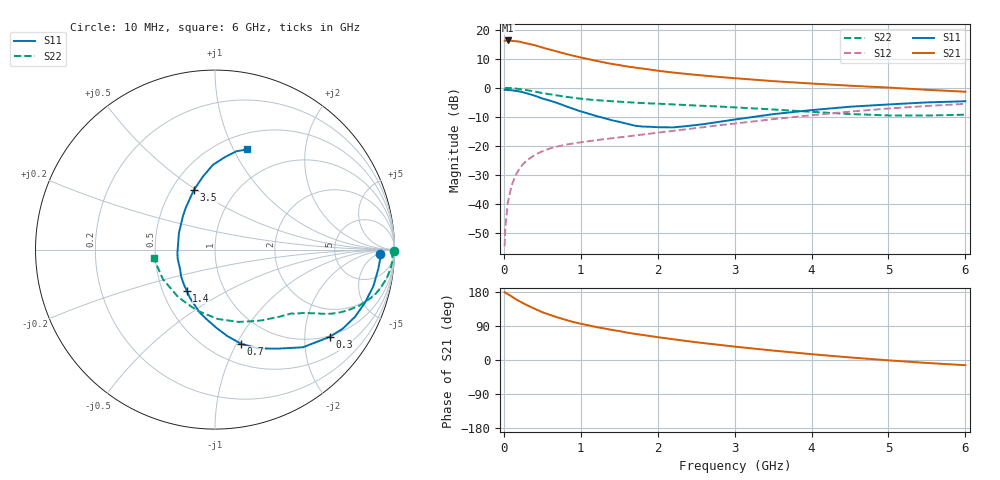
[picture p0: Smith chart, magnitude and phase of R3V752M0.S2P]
! SIEMENS Small Signal Semiconductors
! BFR181
! Si NPN RF Bipolar Junction Transistor in SOT23
! VCE = 0.75 V  IC = 2 mA
! Common Emitter S-Parameters:  May  1996
# GHz  S  MA  R  50
!  f  S11  S21  S12  S22
! GHz  MAG  ANG  MAG  ANG  MAG  ANG  MAG  ANG
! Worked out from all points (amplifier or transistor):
!   36 points, 10 MHz to 6 GHz, reference 50 ohm
!   highest |S21| = 16.3 dB at 50 MHz (marker M1)
!   |S21| within 3 dB of that: start of sweep to 578.3 MHz
!   unconditionally stable (mu >= 1): 1.459 GHz to 3.723 GHz
!   at 250 MHz: K = 0.24, MSG = 20.9 dB, |S12| = -26.3 dB
!   at 1.4 GHz: K = 0.98, MSG = 12.8 dB, |S12| = -17.4 dB
!   at 6 GHz: K = 0.92, MSG = 2.1 dB, |S12| = -5.5 dB
!   S11 on the Smith chart (normalised r, x): 10 MHz: 22, -7; 300 MHz: 0.97, -2.65; 700 MHz: 0.70, -1.04; 1.4 GHz: 0.66, -0.33; 3.5 GHz: 0.64, +0.49; 6 GHz: 0.67, +1.14
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0.01  0.9215 -1.4  6.427 179.1  0.0019 86.6  0.9949 -0.6
0.02  0.9229 -2.6  6.391 177.4  0.004 90.5  0.9862 -1.3
0.05  0.9164 -6.7  6.498 173.9  0.0104 86.2  0.9919 -3.3
0.1  0.9056 -13.0  6.404 168.1  0.0208 82.3  0.9827 -6.4
0.15  0.8866 -19.4  6.317 161.1  0.0308 78.2  0.9701 -9.4
0.2  0.8655 -25.6  6.21 155.5  0.0401 74.9  0.951 -12.3
0.3  0.8025 -37.3  5.764 144.7  0.0567 68.9  0.9095 -17.2
0.4  0.7325 -48.0  5.399 135.4  0.0701 63.6  0.8612 -21.4
0.5  0.6542 -57.5  4.914 126.1  0.0809 59.3  0.8117 -24.7
0.7  0.5447 -74.5  4.172 112.3  0.0981 53.9  0.7352 -29.1
0.8  0.4857 -82.0  3.833 106.2  0.1047 51.9  0.703 -30.6
0.9  0.4358 -89.0  3.557 100.4  0.1105 51.1  0.6733 -31.9
1.1  0.3599 -103.9  3.105 91.4  0.1205 49.8  0.6298 -34.2
1.2  0.3275 -110.5  2.905 87.1  0.1258 49.3  0.6136 -35.2
1.4  0.2777 -124.7  2.571 79.6  0.1354 49.2  0.5877 -37.2
1.7  0.2236 -150.5  2.229 69.2  0.151 50.1  0.5549 -39.9
2.2  0.2086 169.5  1.826 54.8  0.1817 51.1  0.5181 -46.3
2.8  0.2599 133.2  1.535 40.0  0.227 50.7  0.4758 -55.8
3.5  0.3522 109.6  1.3 24.9  0.2887 47.5  0.4237 -72.0
4.5  0.4726 91.4  1.085 6.8  0.3894 38.6  0.3534 -106.9
5.5  0.5603 77.8  0.923 -7.8  0.4866 26.2  0.3336 -150.4
6  0.5866 72.1  0.855 -13.7  0.5294 19.1  0.3445 -171.9
